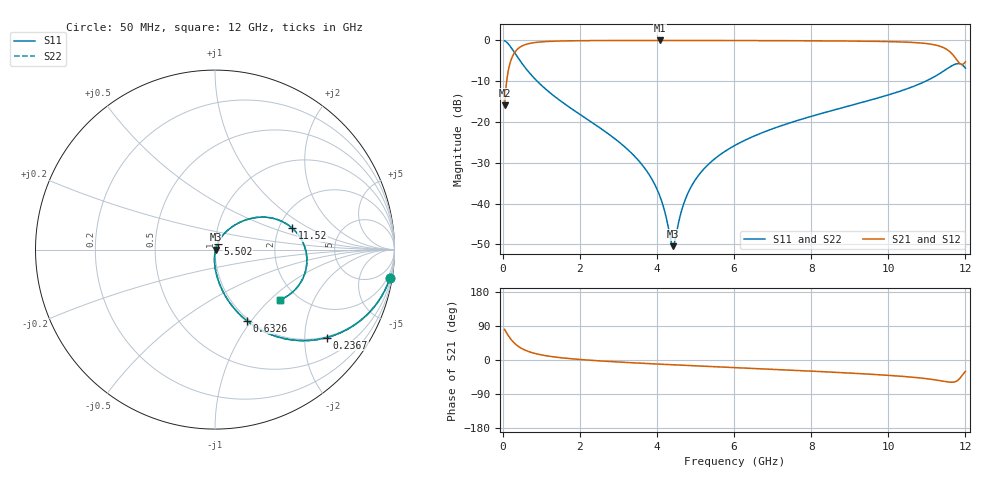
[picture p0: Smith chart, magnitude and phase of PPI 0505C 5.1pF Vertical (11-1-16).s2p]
# GHz S MA R 50
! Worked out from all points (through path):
!   1601 points, 50 MHz to 12 GHz, reference 50 ohm
!   highest |S21| = -0.03 dB at 4.068 GHz (marker M1); lowest = -16.0 dB at 50 MHz (marker M2)
!   group delay of S21, straight-line fit = 17.7 ps
!   lowest |S11| = -50.5 dB at 4.412 GHz (marker M3), VSWR 1.01, Z = 50.3 - j0.0775 ohm
!   |S11| at or under -10 dB: 893 MHz to 10.97 GHz (10.08 GHz wide, 170 % of centre)
!   |S22| runs from -50.5 to -0.1 dB; largest |S21 - S12| = 0
!   S11 on the Smith chart (normalised r, x): 50 MHz: 1, -12; 236.7 MHz: 0.97, -2.57; 632.6 MHz: 0.97, -0.95; 5.502 GHz: 1.03, +0.07; 11.52 GHz: 2.37, +0.70; 12 GHz: 1.62, -1.15
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0.05  0.9872 -9.3  0.1594 80.7  0.1594 80.7  0.9872 -9.3
0.1470937  0.903 -25.8  0.4292 64.1  0.4292 64.1  0.903 -25.8
0.2367188  0.7935 -38.1  0.608 51.8  0.608 51.8  0.7935 -38.1
0.4159687  0.5937 -54.7  0.8038 35.2  0.8038 35.2  0.5937 -54.7
0.6325625  0.4326 -66.0  0.9004 23.8  0.9004 23.8  0.4326 -66.0
1.110562  0.2537 -78.2  0.9657 11.5  0.9657 11.5  0.2537 -78.2
2.044156  0.1201 -88.0  0.9906 1.0  0.9906 1.0  0.1201 -88.0
3.366125  0.04036 -93.7  0.9964 -7.3  0.9964 -7.3  0.04036 -93.7
3.7545  0.02432 -92.9  0.9967 -9.4  0.9967 -9.4  0.02432 -92.9
4.038312  0.01369 -88.8  0.9968 -10.8  0.9968 -10.8  0.01369 -88.8
4.068187  0.01262 -87.8  0.9968 -10.9  0.9968 -10.9  0.01262 -87.8
4.41175  0.003001 -14.9  0.9967 -12.6  0.9967 -12.6  0.003001 -14.9
4.665687  0.009014 56.1  0.9966 -13.8  0.9966 -13.8  0.009014 56.1
4.844938  0.01471 62.9  0.9964 -14.7  0.9964 -14.7  0.01471 62.9
5.502187  0.03543 66.7  0.9956 -17.7  0.9956 -17.7  0.03543 66.7
6.025  0.05165 65.8  0.9946 -20.1  0.9946 -20.1  0.05165 65.8
8.019156  0.1176 58.1  0.9875 -29.5  0.9875 -29.5  0.1176 58.1
10.01331  0.2152 46.5  0.9651 -40.6  0.9651 -40.6  0.2152 46.5
10.93944  0.3109 35.6  0.919 -48.7  0.919 -48.7  0.3109 35.6
11.522  0.4474 15.4  0.7715 -57.5  0.7715 -57.5  0.4474 15.4
11.79087  0.5175 -9.2  0.5649 -54.5  0.5649 -54.5  0.5175 -9.2
12  0.4561 -37.9  0.5456 -29.8  0.5456 -29.8  0.4561 -37.9
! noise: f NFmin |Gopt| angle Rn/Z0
0.05  0.0005306  0.9083  1.969  0.00127
1.372  0.004885  0.7261  4.555  0.003538
2.701  0.008019  0.6804  8.072  0.004831
4.031  0.01086  0.6542  11.61  0.005924
5.36  0.01365  0.6389  15.12  0.007016
6.682  0.01662  0.6332  18.56  0.00831
8.012  0.02033  0.6409  22  0.01032
9.341  0.02669  0.6763  25.53  0.01517
10.67  0.0478  0.782  29.41  0.04212
12  0.3067  0.9582  33.47  1.52
